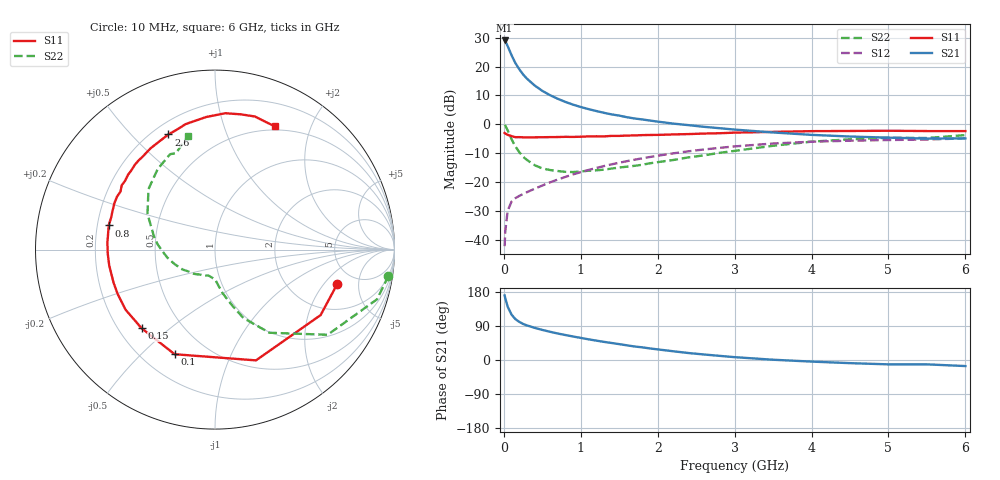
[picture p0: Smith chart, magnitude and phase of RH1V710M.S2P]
! SIEMENS Small Signal Semiconductors
! BFR106
! Si NPN RF Bipolar Junction Transistor in SOT23
! VCE = 1.75 V  IC = 10 mA
! Common Emitter S-Parameters:  August  1996
# GHz  S  MA  R  50
!  f  S11  S21  S12  S22
! GHz  MAG  ANG  MAG  ANG  MAG  ANG  MAG  ANG
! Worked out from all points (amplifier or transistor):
!   36 points, 10 MHz to 6 GHz, reference 50 ohm
!   highest |S21| = 29.0 dB at 10 MHz (marker M1)
!   |S21| within 3 dB of that: start of sweep to 66.38 MHz
!   unconditionally stable (mu >= 1): 470.1 MHz to 2.452 GHz; 4.54 GHz to end of sweep
!   at 250 MHz: K = 0.72, MSG = 20.7 dB, |S12| = -24.1 dB
!   at 1.4 GHz: K = 1.11, MAG = 6.7 dB, |S12| = -13.9 dB
!   at 6 GHz: K = 1.02, MAG = -0.9 dB, |S12| = -4.9 dB
!   S11 on the Smith chart (normalised r, x): 10 MHz: 3.57, -2.77; 100 MHz: 0.33, -0.63; 150 MHz: 0.29, -0.40; 800 MHz: 0.25, +0.11; 2.6 GHz: 0.26, +0.64; 6 GHz: 0.45, +1.50
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0.01  0.7072 -15.9  28.24 170.3  0.0078 84.3  0.9771 -8.6
0.02  0.6924 -31.8  27.27 162.2  0.0147 76.1  0.9448 -17.0
0.05  0.6581 -69.7  22.48 140.6  0.032 60.1  0.7869 -37.1
0.1  0.6248 -111.1  15.71 119.9  0.0461 47.0  0.5536 -56.8
0.15  0.5994 -133.0  11.47 107.8  0.0528 42.9  0.4134 -67.4
0.2  0.6003 -146.1  9.008 100.7  0.0577 42.9  0.3315 -72.5
0.25  0.5961 -155.3  7.306 95.2  0.0623 44.1  0.2746 -77.1
0.3  0.5945 -161.9  6.167 91.3  0.067 46.2  0.2422 -80.5
0.4  0.5959 -171.4  4.705 84.9  0.0768 49.3  0.1967 -85.1
0.5  0.598 -177.7  3.791 79.4  0.0873 52.3  0.1726 -88.7
0.6  0.6008 176.2  3.198 74.5  0.099 54.6  0.162 -92.8
0.7  0.6026 170.9  2.768 69.9  0.1107 55.9  0.1557 -97.2
0.8  0.6076 167.2  2.441 65.9  0.123 56.8  0.1507 -101.7
1.1  0.6175 155.2  1.833 54.6  0.1622 57.7  0.1573 -113.7
1.3  0.6178 148.5  1.583 47.9  0.1894 57.1  0.1642 -122.6
1.6  0.6392 139.3  1.327 38.7  0.2305 54.9  0.1851 -136.0
2.2  0.6686 122.6  1.03 23.1  0.3144 47.8  0.2412 -161.1
2.6  0.6923 112.0  0.906 14.6  0.367 41.7  0.2901 -177.4
3.5  0.7405 93.8  0.723 0.7  0.4654 26.9  0.4256 152.1
4.5  0.7673 79.2  0.615 -8.3  0.5208 10.8  0.5505 125.5
5.5  0.7647 67.9  0.567 -11.5  0.5463 1.0  0.5792 112.1
6  0.7638 64.1  0.571 -16.0  0.5708 -6.1  0.6512 103.2
